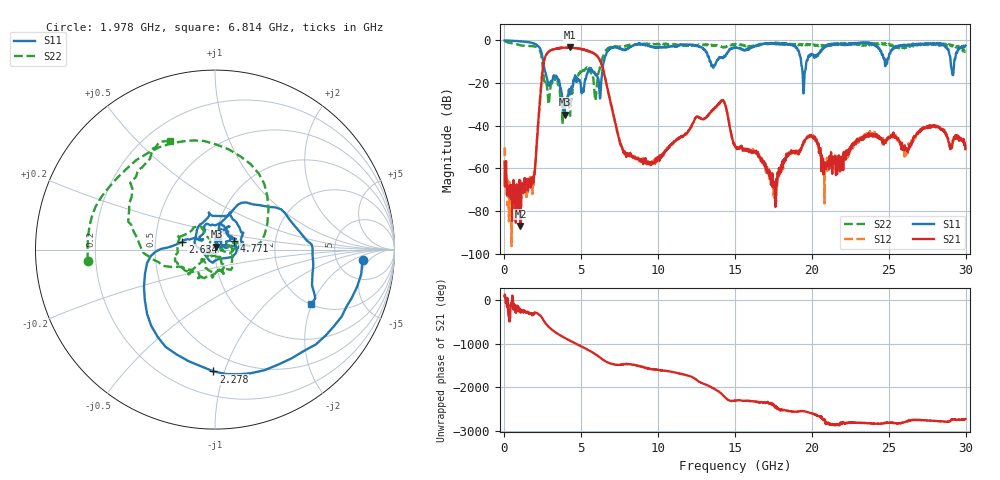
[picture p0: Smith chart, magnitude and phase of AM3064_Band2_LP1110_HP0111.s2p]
# Hz S DB R 50.0
!freq dBS11 angS11 dBS21 angS21 dBS12 angS12 dBS22 angS22
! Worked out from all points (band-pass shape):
!   1600 points, 10 MHz to 29.98 GHz, reference 50 ohm
!   highest |S21| = -3.29 dB at 4.246 GHz (marker M1); lowest = -87.0 dB at 1.041 GHz (marker M2)
!   |S21| within 3 dB of the highest: 2.756 GHz to 5.849 GHz (3.093 GHz wide, 71.9 % of centre)
!   lowest |S11| = -34.8 dB at 3.927 GHz (marker M3), VSWR 1.04, Z = 50.8 + j1.67 ohm
!   |S11| at or under -10 dB: 2.53 GHz to 6.46 GHz (3.93 GHz wide, 87.4 % of centre); 13.42 GHz to 13.79 GHz (373.8 MHz wide, 2.75 % of centre); 19.29 GHz to 19.64 GHz (348.2 MHz wide, 1.79 % of centre)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
!   |S22| runs from -39.3 to -0.3 dB; largest |S21 - S12| = 0.014
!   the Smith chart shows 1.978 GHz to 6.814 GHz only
!   S11 on the Smith chart (normalised r, x): 1.978 GHz: 9.12, -3.35; 2.278 GHz: 0.37, -0.92; 2.634 GHz: 0.69, +0.06; 4.771 GHz: 1.23, +0.12; 6.814 GHz: 2.03, -1.98
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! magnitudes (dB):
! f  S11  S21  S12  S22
! 10 MHz  0.0  -57.1  -50.3  -0.3
! 347.4 MHz  -0.1  -69.7  -71.1  -1.1
! 1.041 GHz  -0.4  -87.0  -67.3  -2.2
! 1.978 GHz  -1.7  -60.9  -61.1  -2.9
! 2.278 GHz  -3.4  -31.0  -31.0  -4.3
! 2.634 GHz  -14.6  -8.1  -8.0  -18.7
! 3.927 GHz  -34.8  -3.4  -3.4  -29.7
! 4.246 GHz  -23.4  -3.3  -3.3  -34.7
! 4.771 GHz  -18.6  -3.8  -3.6  -16.9
! 5.015 GHz  -24.7  -4.1  -4.0  -15.8
! 5.933 GHz  -16.4  -6.7  -6.8  -27.5
! 6.814 GHz  -4.2  -26.4  -26.4  -3.7
! 7.826 GHz  -4.6  -53.0  -52.9  -2.7
! 10 GHz  -3.4  -55.3  -55.5  -1.8
! 14.14 GHz  -8.0  -28.4  -28.3  -2.9
! 15 GHz  -3.2  -49.7  -49.3  -2.0
! 17.59 GHz  -1.3  -72.1  -66.9  -1.1
! 19.47 GHz  -24.1  -47.4  -47.6  -2.3
! 19.99 GHz  -6.4  -45.1  -45.4  -1.7
! 20.87 GHz  -2.6  -58.1  -57.7  -2.7
! 25 GHz  -8.0  -45.7  -45.8  -1.7
! 29.98 GHz  -2.4  -51.0  -51.4  -4.5
